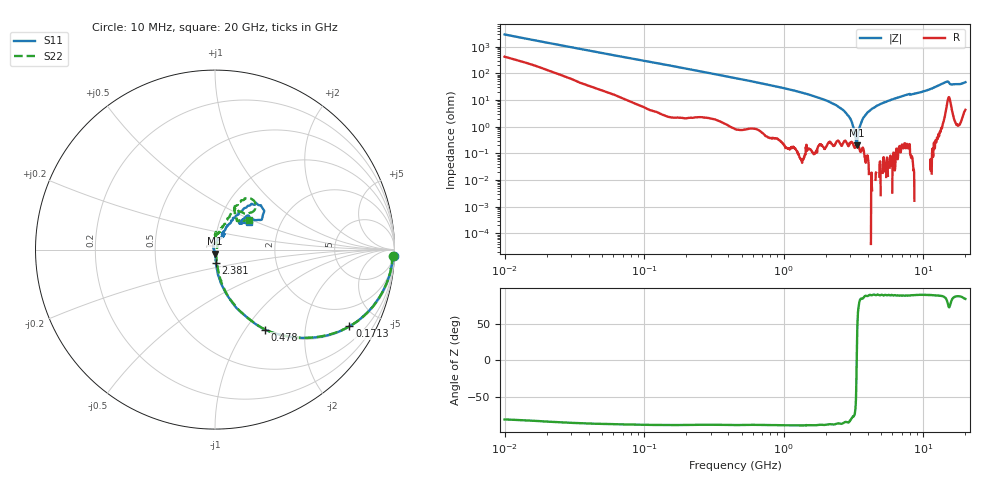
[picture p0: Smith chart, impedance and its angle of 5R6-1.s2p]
!Keysight Technologies,P5008B,MY61100088,A.16.20.02
!Date: Monday, May 27, 2024 16:29:27
!Correction: S11(C* 2-Port  )
!S21(C* 2-Port  )
!S12(C* 2-Port  )
!S22(C* 2-Port  )
!S2P File: Measurements: S11, S21, S12, S22:Log Frequency Sweep
# Hz S  dB  R 50
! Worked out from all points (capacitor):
!   1601 points, 10 MHz to 20 GHz, reference 50 ohm
!   read as one part in series: C = 5.66 pF near 10.39 MHz
!   lowest |Z| = 203 mohm at 3.32 GHz (marker M1)
!   series resonance near 3.329 GHz, so ESL is about 400 pH
!   S11 on the Smith chart (normalised r, x): 10 MHz: 6, -57; 171.3 MHz: 1.04, -3.48; 478 MHz: 1.01, -1.24; 2.381 GHz: 1.00, -0.15; 20 GHz: 1.38, +0.46
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1e7  -0.03 -2.0  -29.14 79.6  -29.15 79.7  -0.06 -2.0
3.555162e7  -0.12 -7.0  -18.17 79.9  -18.18 79.9  -0.13 -7.1
1.263918e8  -0.78 -23.1  -8.17 66.1  -8.19 66.2  -0.77 -23.1
1.71301e8  -1.28 -29.7  -6.15 59.6  -6.16 59.6  -1.28 -29.6
4.472136e8  -5.19 -56.2  -1.65 33.2  -1.65 33.2  -5.18 -56.1
4.779682e8  -5.58 -57.9  -1.48 31.5  -1.49 31.5  -5.57 -57.8
7.946125e8  -9.30 -70.0  -0.57 19.6  -0.59 19.6  -9.29 -69.6
1.589917e9  -16.39 -82.2  -0.10 7.9  -0.11 7.9  -16.30 -80.4
2.380902e9  -22.42 -85.1  -0.02 2.8  -0.03 2.8  -22.22 -81.4
2.934404e9  -27.50 -87.5  -0.00 0.3  -0.01 0.3  -27.68 -80.3
3.32018e9  -32.71 -90.9  0.01 -1.1  -0.00 -1.2  -33.64 -66.0
3.582383e9  -38.42 -106.8  0.01 -2.1  -0.00 -2.1  -39.55 -34.9
3.810595e9  -43.59 -167.0  0.01 -2.8  -0.00 -2.9  -39.00 19.3
4.478574e9  -33.46 114.0  0.01 -4.9  0.00 -4.9  -31.93 59.9
5.652411e9  -26.14 79.5  0.01 -8.0  -0.00 -8.0  -26.22 82.6
7.697294e9  -20.30 59.6  -0.01 -13.1  -0.02 -13.1  -20.57 86.6
8.344716e9  -21.45 58.7  0.01 -14.3  -0.00 -14.4  -21.52 86.1
9.854205e9  -20.09 66.8  -0.00 -18.0  -0.01 -18.1  -20.12 76.0
1.447892e10  -9.21 48.2  -0.79 -31.3  -0.80 -31.4  -9.23 56.0
1.569675e10  -11.42 39.6  -0.83 -26.6  -0.84 -26.7  -11.85 55.6
1.810106e10  -13.58 48.2  -0.23 -33.9  -0.24 -33.9  -13.54 54.6
2e10  -12.14 39.2  -0.58 -39.1  -0.59 -39.2  -11.91 41.1
